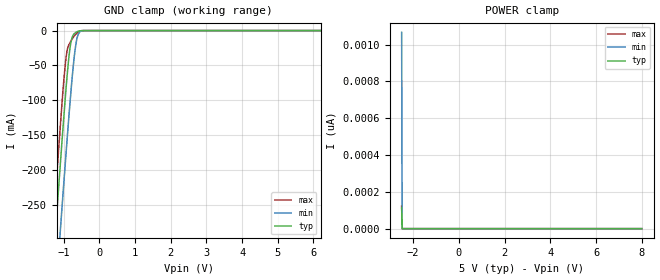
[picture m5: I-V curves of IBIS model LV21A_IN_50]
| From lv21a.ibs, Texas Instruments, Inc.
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|   Model LV21A_IN_50
[Model]   LV21A_IN_50
Model_type   Input
Vinl = 1.5
Vinh = 3.5
|   typ   min   max
C_comp   3.5pF   3.4pF   3.7pF
[Voltage Range]   5   4.5   5.5
[Temperature Range]   25   125   -40
[Power Clamp Reference]   5   4.5   5.5
[GND Clamp Reference]   0   0   0
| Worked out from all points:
|   GND clamp passes 1 mA (typ) near -0.59 V on its own axis
[GND Clamp]
|   Voltage   I(typ)   I(min)   I(max)
-2.5V     -1.244A    -1.327A    -1.203A
-1.303V   -342.6mA   -437mA     -288.7mA
-1.23V    -289mA     -383.9mA   -234.5mA
-1.135V   -220.9mA   -316.2mA   -166mA
-1.072V   -176.4mA   -271.7mA   -121.6mA
-998.5mV  -125.8mA   -220.4mA   -72.97mA
-914.5mV  -71.44mA   -163.3mA   -31.85mA
-799mV    -17.49mA   -89.06mA   -15.38mA
-704.5mV  -4.594mA   -38.07mA   -7.858mA
-631mV    -1.797mA   -12.21mA   -3.542mA
-442mV    -17.94uA   -111.5uA   -18.13uA
8V        0A         0A         0A
[POWER Clamp]
|   Voltage   I(typ)   I(min)   I(max)
-2.5V     113.6pA    1.066nA    123.3pA
-2.479V   0A         0A         0A
-2.469V   0A         0A         0A
8V        0A         0A         0A
